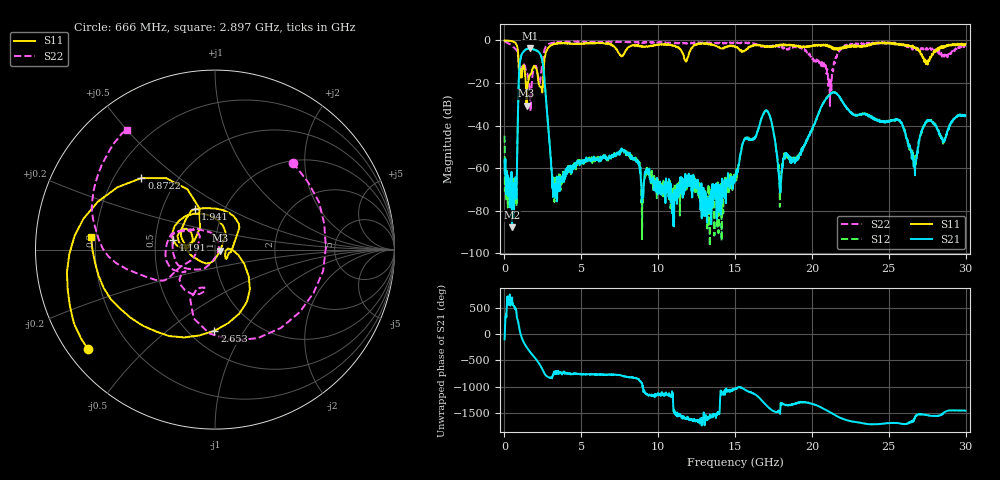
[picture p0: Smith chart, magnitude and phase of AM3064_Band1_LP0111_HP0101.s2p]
# Hz S DB R 50.0
!freq dBS11 angS11 dBS21 angS21 dBS12 angS12 dBS22 angS22
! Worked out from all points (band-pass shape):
!   1600 points, 10 MHz to 29.98 GHz, reference 50 ohm
!   highest |S21| = -3.79 dB at 1.659 GHz (marker M1); lowest = -87.8 dB at 497.3 MHz (marker M2)
!   |S21| within 3 dB of the highest: 1.108 GHz to 2.351 GHz (1.243 GHz wide, 71.9 % of centre)
!   lowest |S11| = -30.7 dB at 1.435 GHz (marker M3), VSWR 1.06, Z = 52.9 - j0.542 ohm
!   |S11| at or under -10 dB: 917 MHz to 2.587 GHz (1.67 GHz wide, 95.3 % of centre); 27.39137 GHz to 27.46003 GHz (68.66 MHz wide, 0.25 % of centre); 27.48882 GHz to 27.56472 GHz (75.9 MHz wide, 0.276 % of centre)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
!   |S22| runs from -33.4 to -0.3 dB; largest |S21 - S12| = 0.01
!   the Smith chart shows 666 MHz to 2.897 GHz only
!   S11 on the Smith chart (normalised r, x): 666 MHz: 0.06, -0.35; 872.2 MHz: 0.31, +0.37; 1.191 GHz: 0.62, +0.07; 1.941 GHz: 0.73, +0.35; 2.653 GHz: 0.66, -0.75; 2.897 GHz: 0.18, +0.05
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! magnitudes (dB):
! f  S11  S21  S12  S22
! 10 MHz  0.0  -56.4  -44.7  -0.3
! 497.3 MHz  -0.4  -87.8  -67.1  -2.6
! 666 MHz  -0.9  -68.5  -67.3  -3.7
! 872.2 MHz  -4.9  -36.0  -36.0  -6.6
! 1.191 GHz  -12.4  -5.7  -5.7  -11.7
! 1.435 GHz  -30.7  -4.1  -4.0  -15.6
! 1.659 GHz  -16.3  -3.8  -3.8  -25.7
! 1.941 GHz  -12.0  -4.4  -4.3  -12.8
! 2.653 GHz  -6.9  -22.7  -22.7  -3.4
! 2.897 GHz  -3.2  -45.0  -44.8  -1.6
! 3.271 GHz  -1.6  -68.3  -69.1  -1.0
! 5.015 GHz  -1.6  -57.2  -56.9  -0.7
! 10 GHz  -2.1  -66.5  -69.2  -0.9
! 15 GHz  -3.0  -64.8  -63.0  -1.4
! 16.97 GHz  -2.7  -33.2  -33.2  -2.9
! 17.95 GHz  -2.4  -71.5  -72.1  -2.7
! 19.99 GHz  -2.8  -41.9  -42.3  -8.2
! 21.4 GHz  -3.6  -24.4  -24.4  -13.2
! 25 GHz  -1.0  -38.1  -37.9  -1.2
! 26.68 GHz  -3.1  -58.4  -57.1  -4.1
! 27.49 GHz  -10.0  -38.1  -37.8  -4.1
! 29.98 GHz  -1.7  -35.2  -35.2  -2.9
